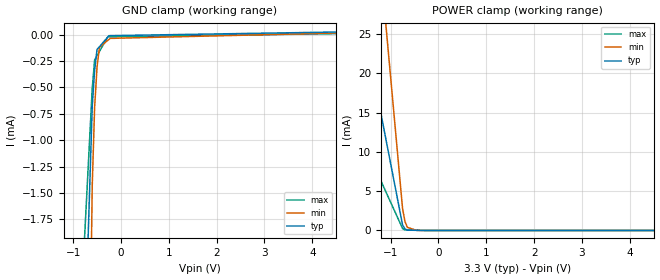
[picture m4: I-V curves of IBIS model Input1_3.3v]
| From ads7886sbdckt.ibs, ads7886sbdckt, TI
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[Model] Input1_3.3v
Model_type Terminator
C_comp 1.513pF 1.513pF 1.513pF
| variable typ   min   max
[Voltage Range] 3.30000V 3.00000V 3.60000V
[POWER Clamp Reference] 3.30000V 3.00000V 3.60000V
[GND Clamp Reference] 0.00000V 0.00000V 0.00000V
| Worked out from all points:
|   POWER clamp passes 1 mA (typ) near -0.76 V on its own axis
[GND Clamp]
-3.3V     -39.67mA   -92.39mA   -24.3mA
-600mV    -681.1uA   -1.428mA   -510uA
-550mV    -338.6uA   -688.2uA   -238.9uA
-500mV    -141.3uA   -310.5uA   -199.3uA
-450mV    -115uA     -120.1uA   -159.7uA
-275mV    -23.06uA   -54.62uA   -21.19uA
-250mV    -9.926uA   -45.26uA   -21.03uA
-225mV    -9.746uA   -35.91uA   -20.87uA
6.6V      39.57uA    37.97uA    22.1uA
[POWER Clamp]
-3.3V     80.72mA    174.1mA    34.44mA
-1.05V    10.12mA    22.94mA    4.277mA
-750mV    705.6uA    2.792mA    255.3uA
-700mV    202.8uA    1.152mA    71.9uA
-650mV    47.18uA    402.4uA    64.71uA
-450mV    18.15uA    40.6pA     35.95uA
6.6V      0A         0A         0A
